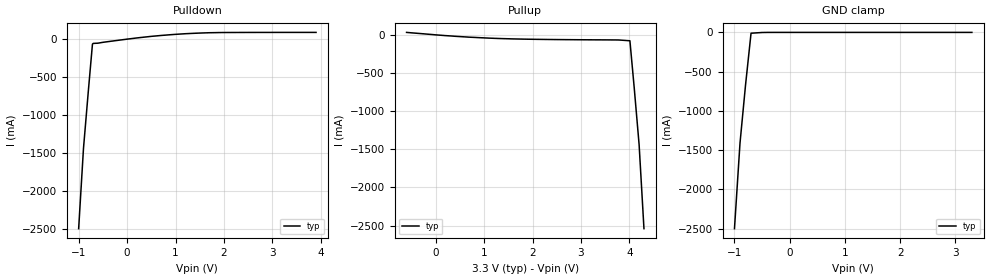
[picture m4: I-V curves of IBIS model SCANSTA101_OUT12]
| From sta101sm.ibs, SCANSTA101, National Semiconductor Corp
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|   3-State Output 12mA MODEL
[Model]   SCANSTA101_OUT12
Model_type   3-state
| Variable   typ   min   max
C_comp   5.00pF   NA   NA
|   typ   min   max
[Temperature Range]   25.0   NA   NA
[Voltage range]   3.3V   NA   NA
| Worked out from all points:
|   slope of the pulldown table from 0 to 0.495 V, typ, clamps not added: 13.6 ohm
|   slope of the pullup table from 0 to 0.495 V, typ, clamps not added: 21.9 ohm
|   GND clamp passes 1 mA (typ) near -0.47 V on its own axis
[Pulldown]
| Voltage   I(typ)   I(min)   I(max)
-1V       -2.5A      NA         NA
-900mV    -1.44A     NA         NA
-800mV    -684mA     NA         NA
-715mV    -65.83mA   NA         NA
-700mV    -56.48mA   NA         NA
500mV     36.8mA     NA         NA
1.3V      74.63mA    NA         NA
2V        87.5mA     NA         NA
3.9V      89mA       NA         NA
[Pullup]
| Voltage   I(typ)   I(min)   I(max)
-600mV    32.15mA    NA         NA
400mV     -18.68mA   NA         NA
1.3V      -47.73mA   NA         NA
3.765V    -66.99mA   NA         NA
4.01V     -77.88mA   NA         NA
4.1V      -702mA     NA         NA
4.2V      -1.44A     NA         NA
4.3V      -2.54A     NA         NA
[GND_clamp]
| Outputs in Tri-state
| Voltage   I(typ)   I(min)   I(max)
-1V       -2.5A      NA         NA
-900mV    -1.41A     NA         NA
-800mV    -672mA     NA         NA
-700mV    -10.6mA    NA         NA
-400mV    -203uA     NA         NA
3.3V      492pA      NA         NA
[POWER_clamp]
| Voltage   I(typ)   I(min)   I(max)
-3.3V     0A         NA         NA
3.3V      0A         NA         NA
[Ramp]
|   typ   min   max
dV/dt_r   1.889/1.60n   NA   NA
dV/dt_f   1.889/0.90n   NA   NA
|[Cload] = 30pF
R_load = 500ohms
